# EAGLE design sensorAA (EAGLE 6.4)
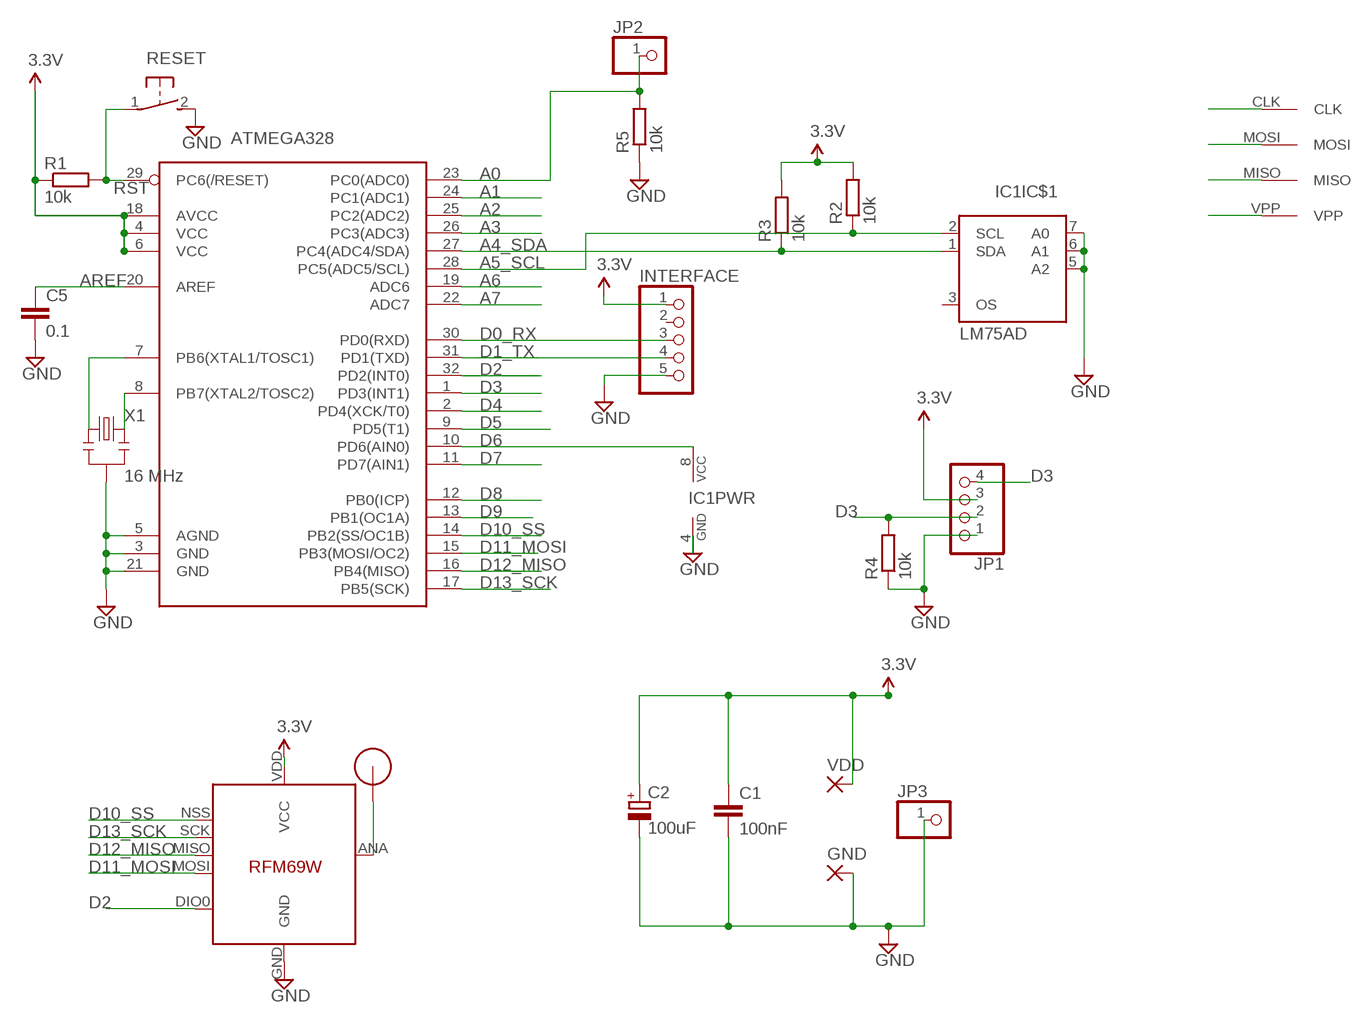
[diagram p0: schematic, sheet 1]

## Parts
ATMEGA328  ATMega-328  ATMEGA168/328TQFP32  [TQFP32-08]
C1  100nF  C-EUC2012  [C2012]
C2  100uF  CPOL-EUSMCB  [SMC_B]
C5  0.1  C-EUC2012  [C2012]
GND  SMD5  [SMD2,54-5,08]
IC1  LM75AD  [SO08]
IC4  RFM69  [RFM69W-MINPADS]
INTERFACE  PINHD-1X05_2.54-S  [1X05-S]
JP1  PINHD-1X04_2.54-S  [1X04-S]
JP2  PINHD-1X01_2.54  [1X01]
JP3  PINHD-1X01_2.54  [1X01]
R1  10k  R-EU_R2012  [R2012]
R2  10k  R-EU_R2012  [R2012]
R3  10k  R-EU_R2012  [R2012]
R4  10k  R-EU_R2012  [R2012]
R5  10k  R-EU_R2012  [R2012]
RESET  DTSM-3  [DTSM-3]
U$1  RFM12B_ANTENNA  [RFM12B-ANTENNA]
U$2  AVRHEADERDIP  [AVRHEADER]
VDD  SMD5  [SMD2,54-5,08]
X1  16 MHz  RESONATORSMD  [RESONATOR-SMD]

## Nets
A0: ATMEGA328.23(PC0(ADC0)) JP2.1 R5.2
A1: ATMEGA328.24(PC1(ADC1))
A2: ATMEGA328.25(PC2(ADC2))
A3: ATMEGA328.26(PC3(ADC3))
A4_SDA: ATMEGA328.27(PC4(ADC4/SDA)) IC1.1(IC$1:SDA) R3.1
A5_SCL: ATMEGA328.28(PC5(ADC5/SCL)) IC1.2(IC$1:SCL) R2.1
A6: ATMEGA328.19(ADC6)
A7: ATMEGA328.22(ADC7)
AREF: ATMEGA328.20(AREF) C5.1
D0_RX: ATMEGA328.30(PD0(RXD)) INTERFACE.3
D1_TX: ATMEGA328.31(PD1(TXD)) INTERFACE.4
D2: ATMEGA328.32(PD2(INT0)) IC4.DIO0
D3: ATMEGA328.1(PD3(INT1)) JP1.2 JP1.4 R4.2
D4: ATMEGA328.2(PD4(XCK/T0))
D5: ATMEGA328.9(PD5(T1))
D6: ATMEGA328.10(PD6(AIN0)) IC1.8(PWR:VCC)
D7: ATMEGA328.11(PD7(AIN1))
D8: ATMEGA328.12(PB0(ICP))
D9: ATMEGA328.13(PB1(OC1A))
D10_SS: ATMEGA328.14(PB2(SS/OC1B)) IC4.NSS(SEL)
D11_MOSI: ATMEGA328.15(PB3(MOSI/OC2)) IC4.MOSI U$2.MOSI
D12_MISO: ATMEGA328.16(PB4(MISO)) IC4.MISO U$2.MISO
D13_SCK: ATMEGA328.17(PB5(SCK)) IC4.SCK U$2.CLK
GND: ATMEGA328.3(GND) ATMEGA328.5(AGND) ATMEGA328.21(GND) C1.2 C2.- C5.2 GND.1(P) IC1.4(PWR:GND) IC1.5(IC$1:A2) IC1.6(IC$1:A1) IC1.7(IC$1:A0) IC4.GND INTERFACE.5 JP1.1 JP3.1 R4.1 R5.1 RESET.2 X1.2
N$1: ATMEGA328.7(PB6(XTAL1/TOSC1)) X1.1
N$3: IC4.ANA(ANT) U$1.P$1
N$21: ATMEGA328.8(PB7(XTAL2/TOSC2)) X1.3
RST: ATMEGA328.29(PC6(/RESET)) R1.2 RESET.1 U$2.VPP
VCC: ATMEGA328.4(VCC) ATMEGA328.6(VCC) ATMEGA328.18(AVCC) C1.1 C2.+ IC4.VDD(VCC) INTERFACE.1 JP1.3 R1.1 R2.2 R3.2 VDD.1(P) ; supply symbol labelled 3.3V
Unconnected: IC1.3(IC$1:OS) INTERFACE.2

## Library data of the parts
ATMEGA328 = LowPowerLab:ATMEGA168/328: Atmel 32-pin 8-bit micro, 16k flash.
C1 C5 = resistor:C-EU: CAPACITOR, European symbol
C2 = resistor:CPOL-EU: POLARIZED CAPACITOR, European symbol
GND VDD = wirepad:SMD5: SMD PAD
IC1 = i2c:LM75AD: Digital Temperature Sensor and Thermal Watchdog
IC4 = LowPowerLab:RFM69
INTERFACE = pinhead-2:PINHD-1X05: PIN HEADER
JP1 = pinhead-2:PINHD-1X04: PIN HEADER
JP2 JP3 = pinhead-2:PINHD-1X01: PIN HEADER
R1-R5 = resistor:R-EU_: RESISTOR, European symbol
RESET = switch-tact:DTSM-3
U$1 = LowPowerLab:RFM12B_ANTENNA
U$2 = RemoteHome:AVRHEADER
X1 = SparkFun:RESONATOR: Resonator Small SMD resonator. This is the itty bitty 10/20MHz resonators with built in caps. CSTCE10M0G55 and CSTCE20M0V53. Footprint has been reviewed closely but hasn't been tested yet.

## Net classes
1 power: width 0.381 mm, clearance 0.254 mm

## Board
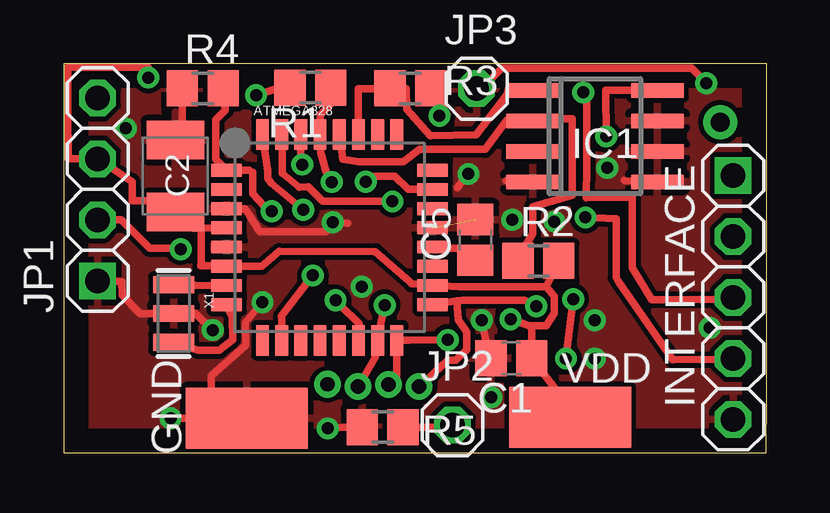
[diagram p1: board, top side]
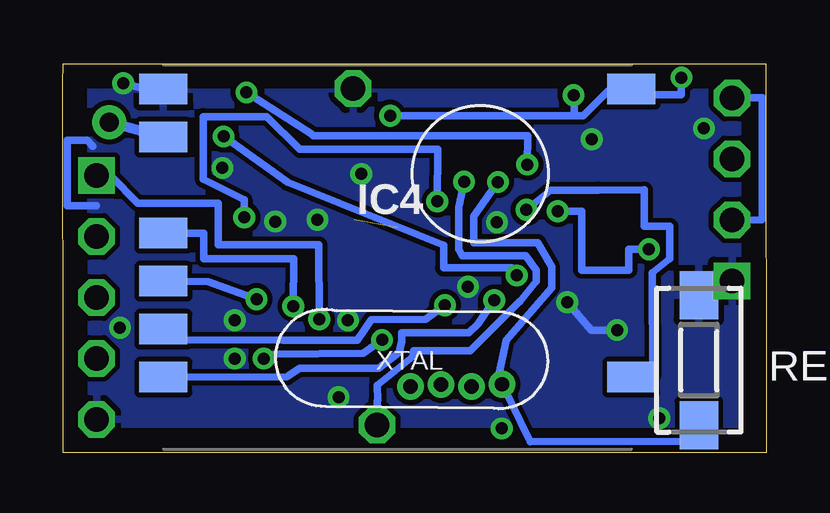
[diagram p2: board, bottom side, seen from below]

Size 29.29 x 16.2 mm. Coordinates in mm from the lower left corner, seen from the top.
Outline: 0,0 29.28,0 29.29,2.34 29.29,15.39 29.29,16.2 0.01,16.2 0,0
Copper layers (1*16): Top 0.035mm / dielectric 1.5mm / Bottom 0.035mm
Design rules "default": minimum track width 10mil, minimum drill 24mil, track to track 8mil, track to pad 8mil, pad to pad 8mil, via to via 8mil, smd to smd 8mil, copper to edge 40mil, drill to drill 8mil, minimum pad ring 10mil, minimum via ring 8mil, stop-mask expansion 4mil, vias tented up to drill 0mil, thermal gap 10mil

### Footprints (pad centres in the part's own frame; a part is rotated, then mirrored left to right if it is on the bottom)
TQFP32-08 = smd 1.27 x 0.533: 1 -4.293,2.8; 2 -4.293,2; 3 -4.293,1.2; 4 -4.293,0.4; 5 -4.293,-0.4; 6 -4.293,-1.2; 7 -4.293,-2; 8 -4.293,-2.8; 17 4.293,-2.8; 18 4.293,-2; 19 4.293,-1.2; 20 4.293,-0.4; 21 4.293,0.4; 22 4.293,1.2; 23 4.293,2; 24 4.293,2.8 | smd 0.533 x 1.27: 9 -2.8,-4.293; 10 -2,-4.293; 11 -1.2,-4.293; 12 -0.4,-4.293; 13 0.4,-4.293; 14 1.2,-4.293; 15 2,-4.293; 16 2.8,-4.293; 25 2.8,4.293; 26 2,4.293; 27 1.2,4.293; 28 0.4,4.293; 29 -0.4,4.293; 30 -1.2,4.293; 31 -2,4.293; 32 -2.8,4.293
C2012 = smd 1.3 x 1.5: 1 -0.85,0; 2 0.85,0
SMC_B = smd 1.6 x 2.4: + -1.5,0; - 1.5,0
SMD2,54-5,08 = smd 2.54 x 5.08: 1 0,0
SO08 = smd 0.6 x 2.2: 1 -1.905,-2.6; 2 -0.635,-2.6; 3 0.635,-2.6; 4 1.905,-2.6; 5 1.905,2.6; 6 0.635,2.6; 7 -0.635,2.6; 8 -1.905,2.6
RFM69W-MINPADS = smd 2 x 1.27: ANA 8,-5; DIO0 -11.5,5; GND 8,-7; MISO 8,1; MOSI 8,3; NSS 8,5; SCK 8,-1; VDD -11.5,-7
1X05-S = drill 1.016 square: 1 -5.08,0 | drill 1.016 octagon: 2 -2.54,0; 3 0,0; 4 2.54,0; 5 5.08,0
1X04-S = drill 1.016 square: 1 -3.81,0 | drill 1.016 octagon: 2 -1.27,0; 3 1.27,0; 4 3.81,0
1X01 = drill 1.016 octagon: 1 0,0
R2012 = smd 1.3 x 1.5: 1 -0.85,0; 2 0.85,0
DTSM-3 = smd 2 x 1.6: 1 -2.7,0; 2 2.7,0
RFM12B-ANTENNA = drill 0.8 pad 1.422: P$1 0,0
AVRHEADER = drill 0.6 pad 0.813: CLK 2.54,0; MISO 1.27,0.091; MOSI 0,0; VPP -1.27,0.099
RESONATOR-SMD = smd 0.7 x 1.7: 1 -1.2,0; 2 0,0; 3 1.2,0

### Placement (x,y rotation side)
ATMEGA328  11.09,8.96 0 top
C1  18.66,3.93 180 top
C2  4.65,11.52 90 top
C5  17.16,8.86 90 top
GND  7.64,1.42 90 top
IC1  22.14,13.18 270 top
IC4  17.11,8.15 180 bottom
INTERFACE  27.9,6.46 270 top
JP1  1.41,10.96 90 top
JP2  16.2,1.15 0 top
JP3  17.2,15.17 0 top
R1  10.28,15.21 0 top
R2  19.78,7.99 0 top
R3  14.44,15.17 0 top
R4  5.8,15.17 0 top
R5  13.29,1.06 0 top
RESET  2.8,3.85 90 bottom
U$1  27.36,13.77 0 top
U$2  12.27,2.74 0 top
VDD  21.1,1.47 90 top
X1  4.58,5.8 270 top

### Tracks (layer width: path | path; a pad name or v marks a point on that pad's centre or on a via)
A0  (via drill 0.5)
  Top 0.305: ATMEGA328.23 14.35,10.96 13.8,11.51 12.95,11.51 v12.58,11.28 | R5.2 16.12,1.06 JP2.1
  Bottom 0.305: v12.58,11.28 12.79,10.22 12.81,10.09 12.81,8.92 12.81,8.81 12.81,8.47 12.66,8.2 10.01,8.2 9.57,7.6 9.57,7.15 10.27,6.28 10.29,6.28 12.33,4.25 14.69,4.24 14.69,4.02 16.19,2.8 16.18,2.19 16.2,2.16 JP2.1
A4_SDA
  Top 0.305: IC1.1 18.55,15.19 18.49,14.94 17.2,13.23 15.27,13.19 14.3,14.29 14.28,15.15 R3.1 14.03,15.15 12.29,15.15 ATMEGA328.27
A5_SCL
  Top 0.305: ATMEGA328.28 11.5,13.24 11.64,12.23 12.3,12.12 14.16,12.12 14.83,12.65 17.56,12.63 18.45,13.85 IC1.2 18.84,13.91 21.18,13.91 21.18,10.73 19.54,10.24 19.54,9.13 18.92,8.09 R2.1
AREF
  Top 0.305: ATMEGA328.20 15.43,8.51 16.41,8.51 17.01,7.91 C5.1
D0_RX  (via drill 0.5)
  Top 0.305: ATMEGA328.30 9.89,12.22 v9.95,12 | v21.65,15.01 21.8,15.01 21.79,14.23 21.79,12.05 21.79,11.93 21.77,10.61 23.7,10.64 23.69,7.71 24.51,6.37 | 24.99,6.37 24.51,6.37 | 24.51,6.37 27.17,6.39 INTERFACE.3
  Bottom 0.305: v9.95,12 9.93,13.21 10.24,13.2 18.86,13.2 18.95,13.29 v21.65,15.01
D1_TX  (via drill 0.5)
  Top 0.305: v13.7,10.46 10.8,10.46 10.18,11.08 9.83,11.05 9.11,11.63 9.1,13.24 ATMEGA328.31 | v21.74,9.79 23.02,9.75 23.03,7.3 23.11,7.14 25.39,3.86 27.2,3.89 INTERFACE.4
  Bottom 0.305: v13.7,10.46 13.7,10.51 13.69,10.52 13.68,12.63 19.43,12.63 20.8,14 23.46,14 23.45,11.38 21.74,10.53 v21.74,9.79
D2  (via drill 0.5)
  Top 0.305: ATMEGA328.32 8.5,11.75 8.51,11.44 8.65,11.22 v9.99,10.11
  Bottom 0.305: v9.99,10.11 8.96,10.94 7.01,10.94 6.99,10.93 5.07,10.95 5.07,9.43 4,9.43 4.01,8.07 4.74,7.5 4.72,3.17 IC4.DIO0
D3  (via drill 0.5)
  Top 0.305: v8.68,10.06 8.61,9.99 7.87,10.79 7.87,11.68 7.74,11.77 ATMEGA328.1 6.34,12.21 6.34,13.86 6.74,14.26 R4.2 | JP1.2 2.39,9.69 3.58,8.51 4.85,8.51 v4.88,8.48
  Bottom 0.305: v8.68,10.06 7.69,10.06 7.68,9.57 7.68,7.6 5.71,7.6 5.72,8.48 v4.88,8.48 | JP1.4 0.16,14.77 0.15,14.78 0.15,9.71 0.18,9.7 JP1.2
D6  (via drill 0.5)
  Top 0.305: IC1.8 22.6,15.09 v22.6,13.17 | v10.38,7.38 9.07,5.69 9.09,5.64 ATMEGA328.10
  Bottom 0.305: v22.6,13.17 22.13,12.84 19.94,11.25 13.44,8.64 13.44,7.69 11.38,7.69 10.6,7.7 v10.38,7.38
D10_SS  (via drill 0.5)
  Top 0.305: v11.33,6.34 11.51,6.17 12.31,5.37 12.33,4.71 ATMEGA328.14
  Bottom 0.305: IC4.NSS 19.96,3.15 19.43,3.51 16.15,3.51 15.28,4.17 15.18,4.65 15.18,4.99 14.65,4.98 14.35,4.99 14.05,4.98 12.38,4.98 12.01,5.35 v11.33,6.34
D11_MOSI  (via drill 0.5)
  Top 0.305: v13.38,6.14 13.06,4.69 ATMEGA328.15 12.99,3.97 U$2.MOSI
  Bottom 0.305: IC4.MOSI 24.34,4.7 20.12,4.68 17.04,4.68 16.44,5.54 14.17,5.54 v13.38,6.14
D12_MISO  (via drill 0.5)
  Top 0.305: v21.23,6.39 v20.93,3.91 | v16,4.69 14.37,4.68 ATMEGA328.16 | U$2.MISO 13.87,3.07 13.89,3.53 ATMEGA328.16 | ATMEGA328.16
  Bottom 0.305: IC4.MISO 23.25,7.11 v21.23,6.39 | v20.93,3.91 20.65,3.92 20.5,4.1 16.78,4.13 v16,4.69
D13_SCK  (via drill 0.5)
  Top 0.305: v19.7,6.1 19.21,6.35 18.56,6.34 16.61,6.35 16.39,6.31 | 16.39,6.31 ATMEGA328.17 | U$2.CLK 16,3.85 16.33,3.85 16.79,4.28 16.8,5.01 16.74,5.12 16.45,5.53 16.39,6.31
  Bottom 0.305: IC4.SCK 23.44,9.15 23.43,8.07 19.69,8.08 v19.7,6.1
GND  (via drill 0.5)  (1 unrouted)
  Top 0.305: IC1.4 18.44,11.33 | ATMEGA328.21 | GND.1 6.24,1.44 5.81,1.44 v4.45,1.43 6.18,1.43 6.18,1.98 6.16,3.2 7.58,4.48 7.56,5.4 v8.28,6.27 | IC1.5 23.38,11.33 23.36,11.35 | ATMEGA328.3 7.54,10.17 7.69,9.97 8.16,9.19 8.9,9.2 10.29,9.2 10.93,9.19 11.33,9.62 v11.21,9.59 11.5,9.57 11.85,9.56 | v6.21,5.11 5.48,5.8 X1.2 3.19,5.79 2.44,6.55 2.43,7.13 JP1.1 | v17.42,5.51 17.67,4.27 C1.2 | v16.87,11.61 16.41,11.03 | R5.1 11.64,1.06 v11.01,1.01 | 4.95,13.05 R4.1 | JP3.1 17.42,15.17 18.26,16.01 26.16,16.01 v26.78,15.39
  Bottom 0.305: IC4.GND 25.83,15.15 v26.78,15.39 | v6.21,5.11 7.28,5.11 v8.28,6.27 | 27.9,10.29 29.11,10.29 29.11,13.01 28.29,13.01 28.05,12.77 | JP1.1 2.92,7.12 RESET.2
  other vias: 18.69,9.7 12.42,6.91 22.65,11.86 20.45,9.62 17.81,2.31 22.13,5.51 22.13,3.92 26.92,5.2 7.26,13.06 2.59,13.5
  pour Top: 0.2,16.05 29.17,16.03 29.1,0.18 0.2,0.22
  pour Bottom: 0.16,16.02 29.12,16.04 29.12,0.15 0.2,0.17
N$1
  Top 0.305: X1.1 5,6.99 5.49,6.97 6.79,6.95 ATMEGA328.7
N$3
  Bottom 0.406: IC4.ANA U$1.P$1
N$21
  Top 0.305: X1.3 5.59,4.26 6.49,4.26 7.04,4.71 7.04,5.62 6.78,6.15 ATMEGA328.8
RST  (via drill 0.5)
  Top 0.305: 10.66,13.28 ATMEGA328.29 | v11.17,11.27 10.95,11.68 10.72,12.5 10.67,13.24 ATMEGA328.29 | R1.2 11.57,14.96 10.69,14.08 ATMEGA328.29
  Bottom 0.305: v11.17,11.27 12.19,9.84 12.19,9.2 12.18,8.75 9.51,8.75 8.94,7.73 8.94,6.87 10.84,4.69 11.12,3.33 11.13,3.05 U$2.VPP 9.83,0.45 2.94,0.47 2.94,1.15 RESET.1
VCC  (via drill 0.5)
  Top 0.305: VDD.1 20.9,1.38 20.93,2.08 | 20.1,2.08 20.93,2.08 | ATMEGA328.4 5.75,9.35 | 5.75,9.35 5.73,9.21 5.73,7.91 5.72,7.77 ATMEGA328.6 8.26,7.76 8.99,8.38 12.98,8.37 14.4,7.14 14.5,7.03 15.34,7 ATMEGA328.18 16.48,6.91 20.1,6.91 | 20.87,7.83 20.68,7.93 R2.2 20.1,6.91 | R3.2 15.98,14.08 v15.66,14.04 | 20.93,2.08 20.68,2.38 C1.1 19.51,5.25 v18.62,5.55 19.41,5.28 20.1,5.28 20.45,5.8 20.45,6.52 20.1,6.91 | 5.75,9.35 5.42,9.35 4.99,9.92 4.52,10.5 4.29,10.5 | 4.29,10.5 2.85,10.49 2.85,11.29 JP1.3 0.19,12.23 0.19,13.2 0.16,13.22 0.16,16.05 3.53,16.05 v3.53,15.63 | 27.89,11.53 INTERFACE.1 | R1.1 8.92,15.19 v8.02,14.89 | C2.+ 4.29,10.14 4.29,10.5
  Bottom 0.305: v15.66,14.04 8.32,14.04 | 8.32,14.04 7.62,14.04 6.59,15.06 5.61,15.06 5.61,15.07 IC4.VDD 4.98,14.9 3.53,14.9 v3.53,15.63 | INTERFACE.1 27.86,11.54 27.86,11.5 27.28,11.5 26.18,10.4 22.82,10.4 22.82,8.66 18.64,8.65 v18.62,5.55 | v8.02,14.89 8,14.04 8.32,14.04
